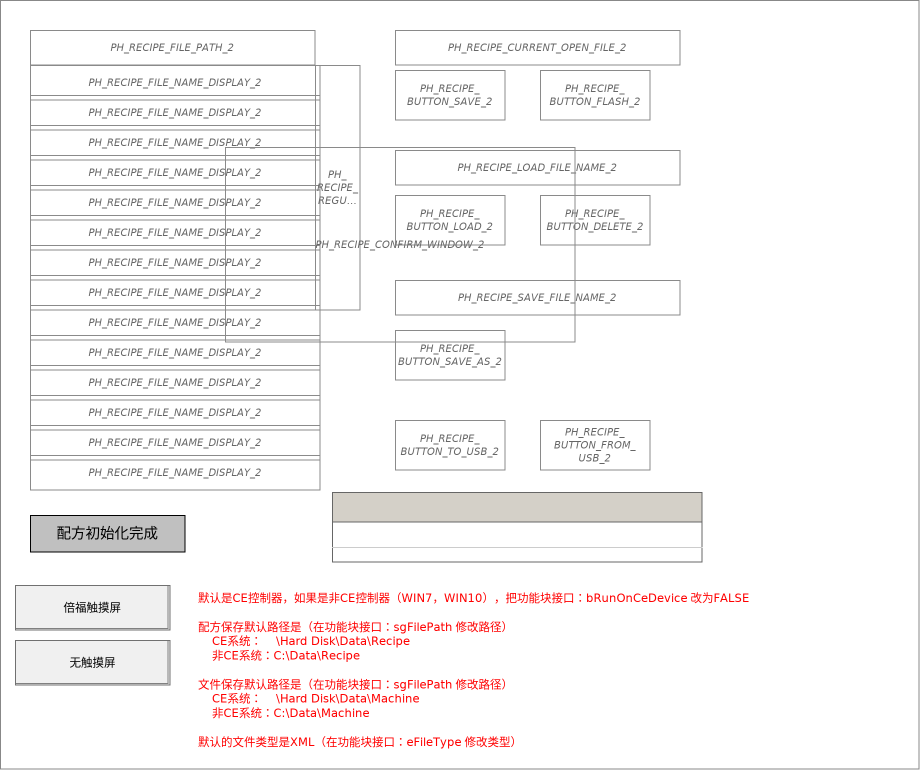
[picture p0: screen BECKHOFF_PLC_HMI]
VISUALIZATION BECKHOFF_PLC_HMI  // 920x770
    RoundedRectangle (30,515 155x37), "配方初始化完成", colour toggle: (Recipe_Manager.g_sRecipeCtrl.sStatus.bInitialOk) <> 0
    Button (15,585 155x45), "倍福触摸屏"
        OnMouseClick: execute { P099_Call_Recipe.iHMI := 1; }
    Rectangle (195,590 725x180), "默认是CE控制器，如果是非CE控制器（WIN7，WIN10），把功能块接口：bRunOnCeDevice 改为FALSE 配方保存默认路径是（在功能块接口：sgFilePath 修改路径） CE系统： \Hard Disk\Data\Recipe 非CE系统：C:\Data\Recipe 文件保存默认路径是（在功能块接口：sgFilePath 修改路径） CE系统： \Hard Disk\Data\Machine 非CE系统：C:\Data\Machine 默认的文件类型是XML（在功能块接口：eFileType 修改类型）"
    Frame (395,195 110x50)
        shows PH_RECIPE_BUTTON_LOAD_2(RECIPE_CTRL_V2 := Recipe_Manager.g_sRecipeCtrl)
        pReferences[0]: m_Input_RECIPE_CTRL_V2=Global_Variables_forRecipe.g_sRecipeCtrl
    Frame (395,330 110x50)
        shows PH_RECIPE_BUTTON_SAVE_AS_2(RECIPE_CTRL_V2 := Recipe_Manager.g_sRecipeCtrl)
        pReferences[0]: m_Input_RECIPE_CTRL_V2=Global_Variables_forRecipe.g_sRecipeCtrl
    Frame (395,70 110x50)
        shows PH_RECIPE_BUTTON_SAVE_2(RECIPE_CTRL_V2 := Recipe_Manager.g_sRecipeCtrl)
        pReferences[0]: m_Input_RECIPE_CTRL_V2=Global_Variables_forRecipe.g_sRecipeCtrl
    Frame (540,70 110x50)
        shows PH_RECIPE_BUTTON_FLASH_2(RECIPE_CTRL_V2 := Recipe_Manager.g_sRecipeCtrl)
        pReferences[0]: m_Input_RECIPE_CTRL_V2=Global_Variables_forRecipe.g_sRecipeCtrl
    Frame (540,195 110x50)
        shows PH_RECIPE_BUTTON_DELETE_2(RECIPE_CTRL_V2 := Recipe_Manager.g_sRecipeCtrl)
        pReferences[0]: m_Input_RECIPE_CTRL_V2=Global_Variables_forRecipe.g_sRecipeCtrl
    Frame (395,420 110x50)
        shows PH_RECIPE_BUTTON_TO_USB_2(RECIPE_CTRL_V2 := Recipe_Manager.g_sRecipeCtrl)
        pReferences[0]: m_Input_RECIPE_CTRL_V2=Global_Variables_forRecipe.g_sRecipeCtrl
    Frame (540,420 110x50)
        shows PH_RECIPE_BUTTON_FROM_USB_2(RECIPE_CTRL_V2 := Recipe_Manager.g_sRecipeCtrl)
        pReferences[0]: m_Input_RECIPE_CTRL_V2=Global_Variables_forRecipe.g_sRecipeCtrl
    Frame (30,30 285x35)
        shows PH_RECIPE_FILE_PATH_2(RECIPE_CTRL_V2 := Recipe_Manager.g_sRecipeCtrl, Right_Edge_Rel := 40)
        pReferences[0]: m_Input_RECIPE_CTRL_V2=Global_Variables_forRecipe.g_sRecipeCtrl, m_Input_Right_Edge_Rel=40
    Frame (395,30 285x35)
        shows PH_RECIPE_CURRENT_OPEN_FILE_2(RECIPE_CTRL_V2 := Recipe_Manager.g_sRecipeCtrl, Right_Edge_Rel := 80)
        pReferences[0]: m_Input_RECIPE_CTRL_V2=Global_Variables_forRecipe.g_sRecipeCtrl, m_Input_Right_Edge_Rel=80
    Frame (395,150 285x35)
        shows PH_RECIPE_LOAD_FILE_NAME_2(RECIPE_CTRL_V2 := Recipe_Manager.g_sRecipeCtrl, Right_Edge_Rel := 80)
        pReferences[0]: m_Input_RECIPE_CTRL_V2=Global_Variables_forRecipe.g_sRecipeCtrl, m_Input_Right_Edge_Rel=80
    Frame (395,280 285x35)
        shows PH_RECIPE_SAVE_FILE_NAME_2(RECIPE_CTRL_V2 := Recipe_Manager.g_sRecipeCtrl, Right_Edge_Rel := 80)
        pReferences[0]: m_Input_RECIPE_CTRL_V2=Global_Variables_forRecipe.g_sRecipeCtrl, m_Input_Right_Edge_Rel=80
    Frame (30,65 290x35)
        shows PH_RECIPE_FILE_NAME_DISPLAY_2(RECIPE_CTRL_V2 := Recipe_Manager.g_sRecipeCtrl, IDX := 1, Right_Edge_Rel := 0)
    Frame (30,95 290x35)
        shows PH_RECIPE_FILE_NAME_DISPLAY_2(RECIPE_CTRL_V2 := Recipe_Manager.g_sRecipeCtrl, IDX := 2, Right_Edge_Rel := 0)
        pReferences[0]: m_Input_RECIPE_CTRL_V2=Global_Variables_forRecipe.g_sRecipeCtrl, m_Input_IDX=2
    Frame (30,125 290x35)
        shows PH_RECIPE_FILE_NAME_DISPLAY_2(RECIPE_CTRL_V2 := Recipe_Manager.g_sRecipeCtrl, IDX := 3, Right_Edge_Rel := 0)
        pReferences[0]: m_Input_RECIPE_CTRL_V2=Global_Variables_forRecipe.g_sRecipeCtrl, m_Input_IDX=3
    Frame (30,155 290x35)
        shows PH_RECIPE_FILE_NAME_DISPLAY_2(RECIPE_CTRL_V2 := Recipe_Manager.g_sRecipeCtrl, IDX := 4, Right_Edge_Rel := 0)
        pReferences[0]: m_Input_RECIPE_CTRL_V2=Global_Variables_forRecipe.g_sRecipeCtrl, m_Input_IDX=4
    Frame (30,185 290x35)
        shows PH_RECIPE_FILE_NAME_DISPLAY_2(RECIPE_CTRL_V2 := Recipe_Manager.g_sRecipeCtrl, IDX := 5, Right_Edge_Rel := 0)
        pReferences[0]: m_Input_RECIPE_CTRL_V2=Global_Variables_forRecipe.g_sRecipeCtrl, m_Input_IDX=5
    Frame (30,215 290x35)
        shows PH_RECIPE_FILE_NAME_DISPLAY_2(RECIPE_CTRL_V2 := Recipe_Manager.g_sRecipeCtrl, IDX := 6, Right_Edge_Rel := 0)
        pReferences[0]: m_Input_RECIPE_CTRL_V2=Global_Variables_forRecipe.g_sRecipeCtrl, m_Input_IDX=6
    Frame (30,245 290x35)
        shows PH_RECIPE_FILE_NAME_DISPLAY_2(RECIPE_CTRL_V2 := Recipe_Manager.g_sRecipeCtrl, IDX := 7, Right_Edge_Rel := 0)
        pReferences[0]: m_Input_RECIPE_CTRL_V2=Global_Variables_forRecipe.g_sRecipeCtrl, m_Input_IDX=7
    Frame (30,275 290x35)
        shows PH_RECIPE_FILE_NAME_DISPLAY_2(RECIPE_CTRL_V2 := Recipe_Manager.g_sRecipeCtrl, IDX := 8, Right_Edge_Rel := 0)
        pReferences[0]: m_Input_RECIPE_CTRL_V2=Global_Variables_forRecipe.g_sRecipeCtrl, m_Input_IDX=8
    Frame (30,305 290x35)
        shows PH_RECIPE_FILE_NAME_DISPLAY_2(RECIPE_CTRL_V2 := Recipe_Manager.g_sRecipeCtrl, IDX := 9, Right_Edge_Rel := 0)
        pReferences[0]: m_Input_RECIPE_CTRL_V2=Global_Variables_forRecipe.g_sRecipeCtrl, m_Input_IDX=9
    Frame (30,335 290x35)
        shows PH_RECIPE_FILE_NAME_DISPLAY_2(RECIPE_CTRL_V2 := Recipe_Manager.g_sRecipeCtrl, IDX := 10, Right_Edge_Rel := 0)
        pReferences[0]: m_Input_RECIPE_CTRL_V2=Global_Variables_forRecipe.g_sRecipeCtrl, m_Input_IDX=10
    Frame (315,65 45x245)
        shows PH_RECIPE_REGULAR(RECIPE_CTRL_V2 := Recipe_Manager.g_sRecipeCtrl)
        pReferences[0]: m_Input_RECIPE_CTRL_V2=Global_Variables_forRecipe.g_sRecipeCtrl
    Frame (30,365 290x35)
        shows PH_RECIPE_FILE_NAME_DISPLAY_2(RECIPE_CTRL_V2 := Recipe_Manager.g_sRecipeCtrl, IDX := 11, Right_Edge_Rel := 0)
        pReferences[0]: m_Input_RECIPE_CTRL_V2=Global_Variables_forRecipe.g_sRecipeCtrl, m_Input_IDX=11
    Frame (30,395 290x35)
        shows PH_RECIPE_FILE_NAME_DISPLAY_2(RECIPE_CTRL_V2 := Recipe_Manager.g_sRecipeCtrl, IDX := 12, Right_Edge_Rel := 0)
        pReferences[0]: m_Input_RECIPE_CTRL_V2=Global_Variables_forRecipe.g_sRecipeCtrl, m_Input_IDX=12
    Frame (30,425 290x35)
        shows PH_RECIPE_FILE_NAME_DISPLAY_2(RECIPE_CTRL_V2 := Recipe_Manager.g_sRecipeCtrl, IDX := 13, Right_Edge_Rel := 0)
        pReferences[0]: m_Input_RECIPE_CTRL_V2=Global_Variables_forRecipe.g_sRecipeCtrl, m_Input_IDX=13
    Frame (30,455 290x35)
        shows PH_RECIPE_FILE_NAME_DISPLAY_2(RECIPE_CTRL_V2 := Recipe_Manager.g_sRecipeCtrl, IDX := 14, Right_Edge_Rel := 0)
        pReferences[0]: m_Input_RECIPE_CTRL_V2=Global_Variables_forRecipe.g_sRecipeCtrl, m_Input_IDX=14
    Frame (225,147 350x195)
        shows PH_RECIPE_CONFIRM_WINDOW_2(RECIPE_CTRL_V2 := Recipe_Manager.g_sRecipeCtrl)
        pReferences[0]: m_Input_RECIPE_CTRL_V2=Global_Variables_forRecipe.g_sRecipeCtrl
    Button (15,640 155x45), "无触摸屏"
        OnMouseClick: execute { P099_Call_Recipe.iHMI := 0; }
    Table (332,492 370x70), data array: sRecData
        p2232123230: rTemp
        p2685023577: sRecData.rTemp
        p3854506369: Global_Variables_Param.sRecData.rTemp
        p511219082: rSpeedRpm
        p3312258591: sRecData.rSpeedRpm
        p1892666644: Global_Variables_Param.sRecData.rSpeedRpm
        p1755163831: rPressure
        p1791247317: sRecData.rPressure
        p338671338: Global_Variables_Param.sRecData.rPressure
        Columns.Column.[2].Template: OnMouseDown: write the text variable via Edit
        Columns.Column.[1].Template: OnMouseDown: write the text variable via Edit
        Columns.Column.[0].Template: OnMouseDown: write the text variable via Edit
END_VISUALIZATION
